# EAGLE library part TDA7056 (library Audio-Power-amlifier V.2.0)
The TDA7056 is a mono output amplifier, designed for battery-fed portable radios and mains-fed equipment such as television. For space reasons there is a trend to decrease the number of external components. For portable applications there is also a trend to decrease the number of battery cells, but still a reasonable output power is required. The TDA7056 fulfills both of these requirements. It needs no peripheral components, because it makes use of the Bridge-Tied-Load (BTL) principle. Consequently it has, at the same supply voltage, a higher output power compared to a conventional Single Ended output stage. It delivers an output power of 1 W into a loudspeaker load of 8 W with 6 V supply or 3 W into 16 W loudspeaker at 11 V without need of an external heatsink. The gain is internally fixed at 40 dB. Special attention is given to switch-on/off click suppression, and it has a good overall stability. The load can be short circuited at all input conditions.
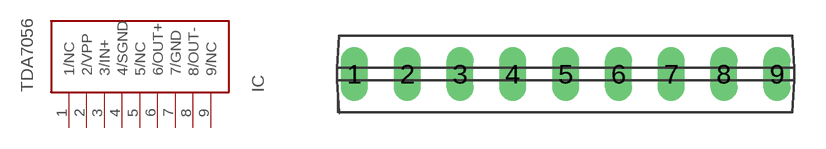
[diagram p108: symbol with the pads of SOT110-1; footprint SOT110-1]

Designator prefix IC

## TDA7056  [SOT110-1]
1  1/NC  nc
2  2/VPP  pwr
3  3/IN+  in
4  4/SGND  pwr
5  5/NC  nc
6  6/OUT+  out
7  7/GND  pwr
8  8/OUT-  out
9  9/NC  nc

## Footprint SOT110-1 (pad centres in mm)
SIL9MPF: plastic single in-line medium power package with fin; 9 leads
drill 0.8 long: 1 -10.16,0; 2 -7.62,0; 3 -5.08,0; 4 -2.54,0; 5 0,0; 6 2.54,0; 7 5.08,0; 8 7.62,0; 9 10.16,0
